FUNCTION "COMANDO USCITE" : VOID
TITLE =COMANDO USCITE
VERSION : 0.1

BEGIN
NETWORK
TITLE =RIPRISTINO EMERGENZA
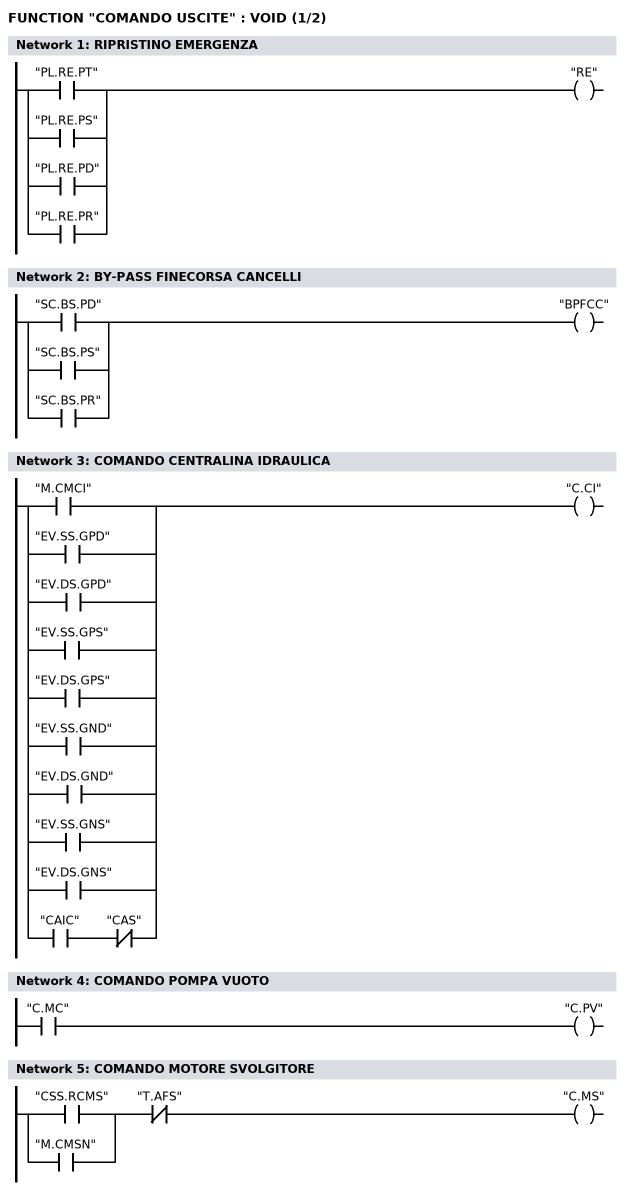
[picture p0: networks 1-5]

      O     "PL.RE.PT";
      O     "PL.RE.PS";
      O     "PL.RE.PD";
      O     "PL.RE.PR";
      =     "RE";
NETWORK
TITLE =BY-PASS FINECORSA CANCELLI

      O     "SC.BS.PD";
      O     "SC.BS.PS";
      O     "SC.BS.PR";
      =     "BPFCC";
NETWORK
TITLE =COMANDO CENTRALINA IDRAULICA

      O     "M.CMCI";
      O     "EV.SS.GPD";
      O     "EV.DS.GPD";
      O     "EV.SS.GPS";
      O     "EV.DS.GPS";
      O     "EV.SS.GND";
      O     "EV.DS.GND";
      O     "EV.SS.GNS";
      O     "EV.DS.GNS";
      O     ;
      U     "CAIC";
      UN    "CAS";
      =     "C.CI";
NETWORK
TITLE =COMANDO POMPA VUOTO

      O     "C.MC";
      =     "C.PV";
NETWORK
TITLE =COMANDO MOTORE SVOLGITORE

      U(    ;
      O     "CSS.RCMS";
      O     "M.CMSN";
      )     ;
      UN    "T.AFS";
      =     "C.MS";
NETWORK
TITLE =COMANDO MOTORE CATENE
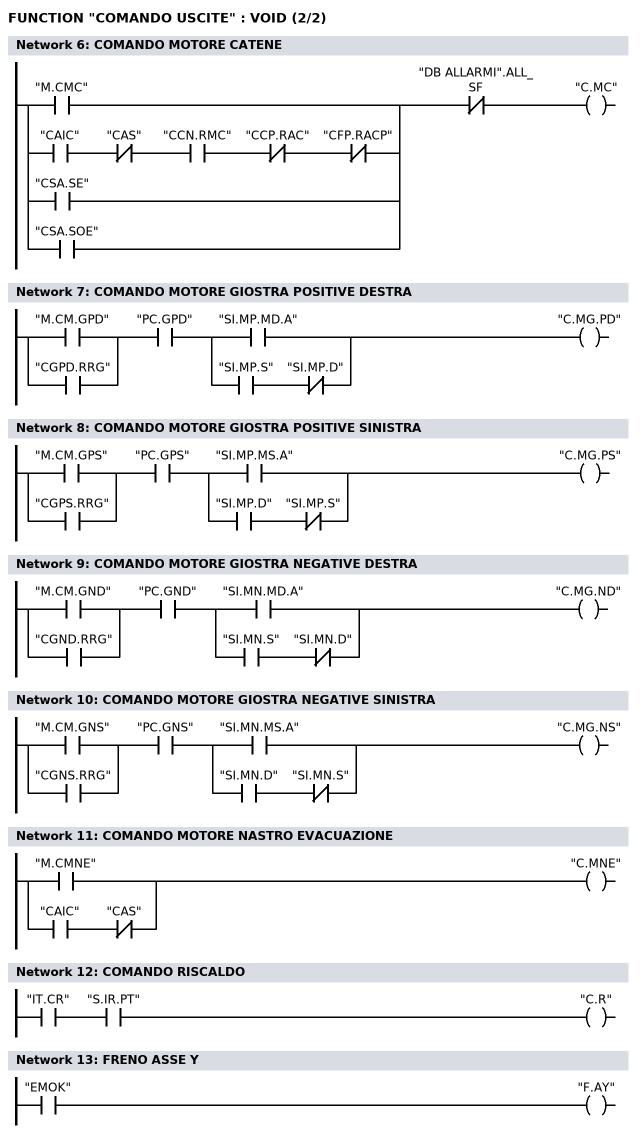
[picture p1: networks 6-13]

      U(    ;
      O     "M.CMC";
      O     ;
      U     "CAIC";
      UN    "CAS";
      U     "CCN.RMC";
      UN    "CCP.RAC";
      UN    "CFP.RACP";
      O     "CSA.SE";
      O     "CSA.SOE";
      )     ;
      UN    "DB ALLARMI".ALL_SF;
      =     "C.MC";
NETWORK
TITLE =COMANDO MOTORE GIOSTRA POSITIVE DESTRA

      U(    ;
      O     "M.CM.GPD";
      O     "CGPD.RRG";
      )     ;
      U     "PC.GPD";
      U(    ;
      O     "SI.MP.MD.A";
      O     ;
      U     "SI.MP.S";
      UN    "SI.MP.D";
      )     ;
      =     "C.MG.PD";
NETWORK
TITLE =COMANDO MOTORE GIOSTRA POSITIVE SINISTRA

      U(    ;
      O     "M.CM.GPS";
      O     "CGPS.RRG";
      )     ;
      U     "PC.GPS";
      U(    ;
      O     "SI.MP.MS.A";
      O     ;
      U     "SI.MP.D";
      UN    "SI.MP.S";
      )     ;
      =     "C.MG.PS";
NETWORK
TITLE =COMANDO MOTORE GIOSTRA NEGATIVE DESTRA

      U(    ;
      O     "M.CM.GND";
      O     "CGND.RRG";
      )     ;
      U     "PC.GND";
      U(    ;
      O     "SI.MN.MD.A";
      O     ;
      U     "SI.MN.S";
      UN    "SI.MN.D";
      )     ;
      =     "C.MG.ND";
NETWORK
TITLE =COMANDO MOTORE GIOSTRA NEGATIVE SINISTRA

      U(    ;
      O     "M.CM.GNS";
      O     "CGNS.RRG";
      )     ;
      U     "PC.GNS";
      U(    ;
      O     "SI.MN.MS.A";
      O     ;
      U     "SI.MN.D";
      UN    "SI.MN.S";
      )     ;
      =     "C.MG.NS";
NETWORK
TITLE =COMANDO MOTORE NASTRO EVACUAZIONE

      O     "M.CMNE";
      O     ;
      U     "CAIC";
      UN    "CAS";
      =     "C.MNE";
NETWORK
TITLE =COMANDO RISCALDO

      U     "IT.CR";
      U     "S.IR.PT";
      =     "C.R";
NETWORK
TITLE =FRENO ASSE Y

      U     "EMOK";
//      UN    "SC.BS.PR"
      =     "F.AY";
NETWORK
TITLE =AGGANCIO FRIZIONE IMBUSTATRICE

      UN(   ;
      O     "M.CAFI";
      O     ;
      U     "CAIC";
      U     "CCP.RAF";
      )     ;
      =     "A.FI";
NETWORK
TITLE =SBLOCCO RIPARI
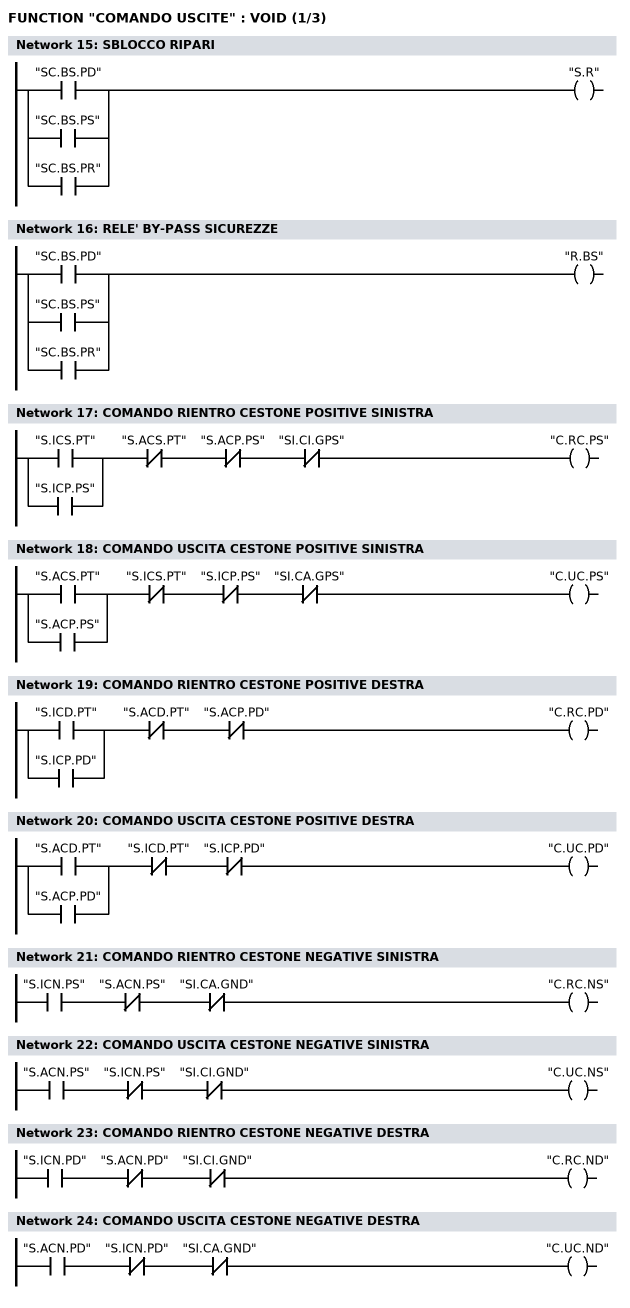
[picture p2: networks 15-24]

      O     "SC.BS.PD";
      O     "SC.BS.PS";
      O     "SC.BS.PR";
      =     "S.R";
NETWORK
TITLE =RELE' BY-PASS SICUREZZE

      O     "SC.BS.PD";
      O     "SC.BS.PS";
      O     "SC.BS.PR";
      =     "R.BS";
NETWORK
TITLE =COMANDO RIENTRO CESTONE POSITIVE SINISTRA

      O     "S.ICS.PT";
      O     "S.ICP.PS";
      UN    "S.ACS.PT";
      UN    "S.ACP.PS";
      UN    "SI.CI.GPS";
      =     "C.RC.PS";
NETWORK
TITLE =COMANDO USCITA CESTONE POSITIVE SINISTRA

      O     "S.ACS.PT";
      O     "S.ACP.PS";
      UN    "S.ICS.PT";
      UN    "S.ICP.PS";
      UN    "SI.CA.GPS";
      =     "C.UC.PS";
NETWORK
TITLE =COMANDO RIENTRO CESTONE POSITIVE DESTRA

      O     "S.ICD.PT";
      O     "S.ICP.PD";
      UN    "S.ACD.PT";
      UN    "S.ACP.PD";
// UN    "SI.CI.GPD"
      =     "C.RC.PD";
NETWORK
TITLE =COMANDO USCITA CESTONE POSITIVE DESTRA

      U     "S.ACD.PT";
      O     "S.ACP.PD";
      UN    "S.ICD.PT";
      UN    "S.ICP.PD";
//  UN    "SI.CA.GPD"
      =     "C.UC.PD";
NETWORK
TITLE =COMANDO RIENTRO CESTONE NEGATIVE SINISTRA

      U     "S.ICN.PS";
      UN    "S.ACN.PS";
      UN    "SI.CA.GND";
      =     "C.RC.NS";
NETWORK
TITLE =COMANDO USCITA CESTONE NEGATIVE SINISTRA

      U     "S.ACN.PS";
      UN    "S.ICN.PS";
      UN    "SI.CI.GND";
      =     "C.UC.NS";
NETWORK
TITLE =COMANDO RIENTRO CESTONE NEGATIVE DESTRA

      U     "S.ICN.PD";
      UN    "S.ACN.PD";
      UN    "SI.CI.GND";
      =     "C.RC.ND";
NETWORK
TITLE =COMANDO USCITA CESTONE NEGATIVE DESTRA

      U     "S.ACN.PD";
      UN    "S.ICN.PD";
      UN    "SI.CA.GND";
      =     "C.UC.ND";
NETWORK
TITLE =COMANDO APERTURA FRENO GIOSTRA POSITIVA DESTRA
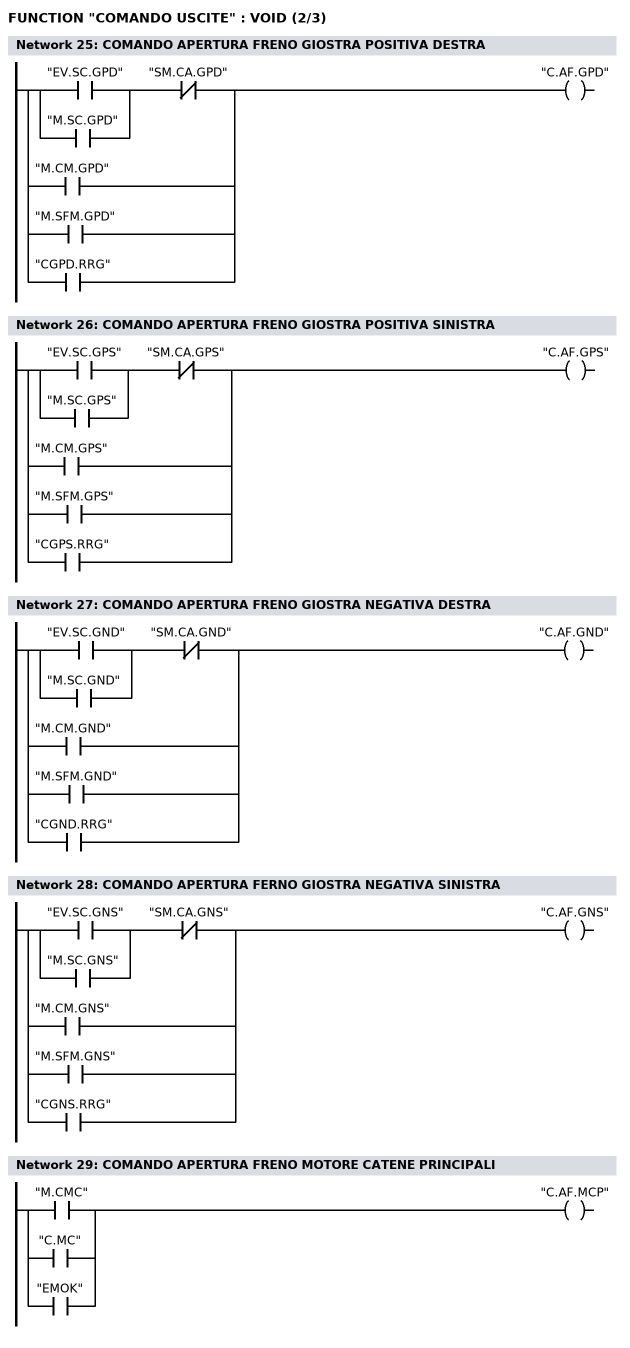
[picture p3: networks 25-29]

      O     "EV.SC.GPD";
      O     "M.SC.GPD";
      UN    "SM.CA.GPD";
      O     ;
      O     "M.CM.GPD";
      O     "M.SFM.GPD";
      O     "CGPD.RRG";
      =     "C.AF.GPD";
NETWORK
TITLE =COMANDO APERTURA FRENO GIOSTRA POSITIVA SINISTRA

      O     "EV.SC.GPS";
      O     "M.SC.GPS";
      UN    "SM.CA.GPS";
      O     ;
      O     "M.CM.GPS";
      O     "M.SFM.GPS";
      O     "CGPS.RRG";
      =     "C.AF.GPS";
NETWORK
TITLE =COMANDO APERTURA FRENO GIOSTRA NEGATIVA DESTRA

      O     "EV.SC.GND";
      O     "M.SC.GND";
      UN    "SM.CA.GND";
      O     ;
      O     "M.CM.GND";
      O     "M.SFM.GND";
      O     "CGND.RRG";
      =     "C.AF.GND";
NETWORK
TITLE =COMANDO APERTURA FERNO GIOSTRA NEGATIVA SINISTRA

      O     "EV.SC.GNS";
      O     "M.SC.GNS";
      UN    "SM.CA.GNS";
      O     ;
      O     "M.CM.GNS";
      O     "M.SFM.GNS";
      O     "CGNS.RRG";
      =     "C.AF.GNS";
NETWORK
TITLE =COMANDO APERTURA FRENO MOTORE CATENE PRINCIPALI

      O     "M.CMC";
      O     "C.MC";
      O     "EMOK";
      =     "C.AF.MCP";
NETWORK
TITLE =COMANDO ABILITAZIONE REGOLATORE ASSE X
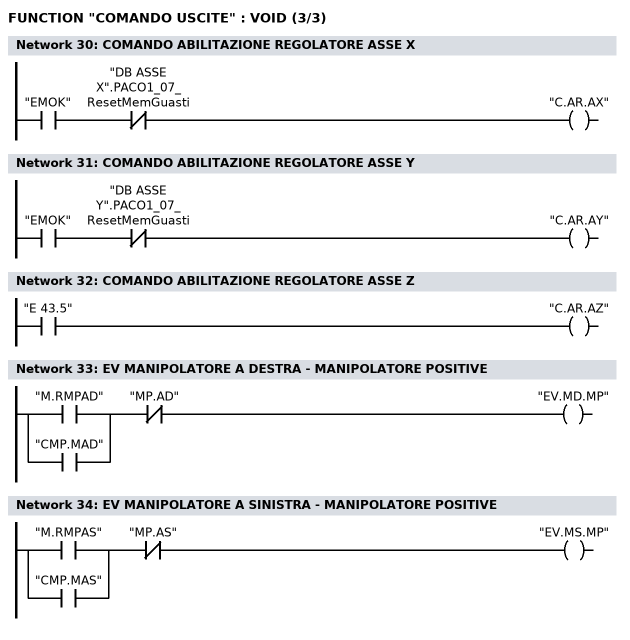
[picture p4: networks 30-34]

      U     "EMOK";
      UN    "DB ASSE X".PACO1_07_ResetMemGuasti;
      =     "C.AR.AX";
NETWORK
TITLE =COMANDO ABILITAZIONE REGOLATORE ASSE Y

      U     "EMOK";
      UN    "DB ASSE Y".PACO1_07_ResetMemGuasti;
      =     "C.AR.AY";
NETWORK
TITLE =COMANDO ABILITAZIONE REGOLATORE ASSE Z

      U     "E      43.5";
      =     "C.AR.AZ";
NETWORK
TITLE =EV MANIPOLATORE A DESTRA - MANIPOLATORE POSITIVE

      O     "M.RMPAD";
      O     "CMP.MAD";
      UN    "MP.AD";
      =     "EV.MD.MP";
NETWORK
TITLE =EV MANIPOLATORE A SINISTRA - MANIPOLATORE POSITIVE

      O     "M.RMPAS";
      O     "CMP.MAS";
      UN    "MP.AS";
      =     "EV.MS.MP";
NETWORK
TITLE =scorta

      CLR   ;
      =     "A      14.2";
NETWORK
TITLE =scorta

      CLR   ;
      =     "A      14.3";
NETWORK
TITLE =EV SALITA MANO DESTRA MANIPOLATORE POSITIVE
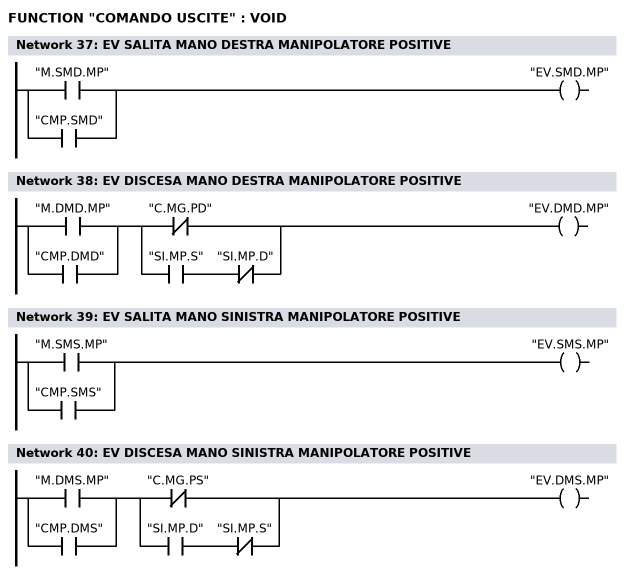
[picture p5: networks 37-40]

      O     "M.SMD.MP";
      O     "CMP.SMD";
      =     "EV.SMD.MP";
NETWORK
TITLE =EV DISCESA MANO DESTRA MANIPOLATORE POSITIVE

      U(    ;
      O     "M.DMD.MP";
      O     "CMP.DMD";
      )     ;
      U(    ;
      ON    "C.MG.PD";
      O     ;
      U     "SI.MP.S";
      UN    "SI.MP.D";
      )     ;
      =     "EV.DMD.MP";
NETWORK
TITLE =EV SALITA MANO SINISTRA MANIPOLATORE POSITIVE

      O     "M.SMS.MP";
      O     "CMP.SMS";
      =     "EV.SMS.MP";
NETWORK
TITLE =EV DISCESA MANO SINISTRA MANIPOLATORE POSITIVE

      U(    ;
      O     "M.DMS.MP";
      O     "CMP.DMS";
      )     ;
      U(    ;
      ON    "C.MG.PS";
      O     ;
      U     "SI.MP.D";
      UN    "SI.MP.S";
      )     ;
      =     "EV.DMS.MP";
NETWORK
TITLE =

      CLR   ;
      =     "A      15.0";
NETWORK
TITLE =

      CLR   ;
      =     "A      15.1";
NETWORK
TITLE =scorta

      CLR   ;
      =     "A      15.2";
NETWORK
TITLE =scorta

      CLR   ;
      =     "A      15.3";
NETWORK
TITLE =LP EMERGENZA
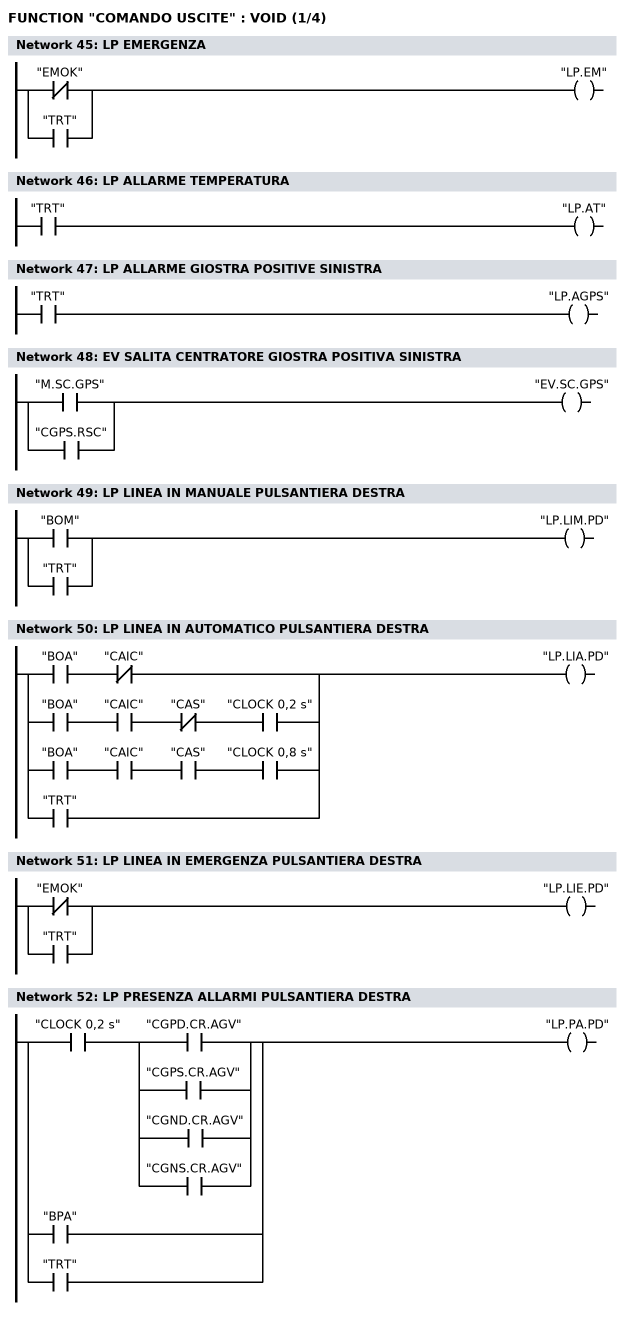
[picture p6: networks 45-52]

      ON    "EMOK";
      O     "TRT";
      =     "LP.EM";
NETWORK
TITLE =LP ALLARME TEMPERATURA

      O     "TRT";
      =     "LP.AT";
NETWORK
TITLE =LP ALLARME GIOSTRA POSITIVE SINISTRA

      O     "TRT";
      =     "LP.AGPS";
NETWORK
TITLE =EV SALITA CENTRATORE GIOSTRA POSITIVA SINISTRA

      O     "M.SC.GPS";
      O     "CGPS.RSC";
      =     "EV.SC.GPS";
NETWORK
TITLE =LP LINEA IN MANUALE PULSANTIERA DESTRA

      O     "BOM";
      O     "TRT";
      =     "LP.LIM.PD";
NETWORK
TITLE =LP LINEA IN AUTOMATICO PULSANTIERA DESTRA

      U     "BOA";
      UN    "CAIC";
      O     ;
      U     "BOA";
      U     "CAIC";
      UN    "CAS";
      U     "CLOCK 0,2 s";
      O     ;
      U     "BOA";
      U     "CAIC";
      U     "CAS";
      U     "CLOCK 0,8 s";
      O     "TRT";
      =     "LP.LIA.PD";
NETWORK
TITLE =LP LINEA IN EMERGENZA PULSANTIERA DESTRA

      ON    "EMOK";
      O     "TRT";
      =     "LP.LIE.PD";
NETWORK
TITLE =LP PRESENZA ALLARMI PULSANTIERA DESTRA

      U     "CLOCK 0,2 s";
      U(    ;
      O     "CGPD.CR.AGV";
      O     "CGPS.CR.AGV";
      O     "CGND.CR.AGV";
      O     "CGNS.CR.AGV";
      )     ;
      O     "BPA";
      O     "TRT";
      =     "LP.PA.PD";
NETWORK
TITLE =LP MARCIA MOTORE GIOSTRA PULSANTIERA DESTRA
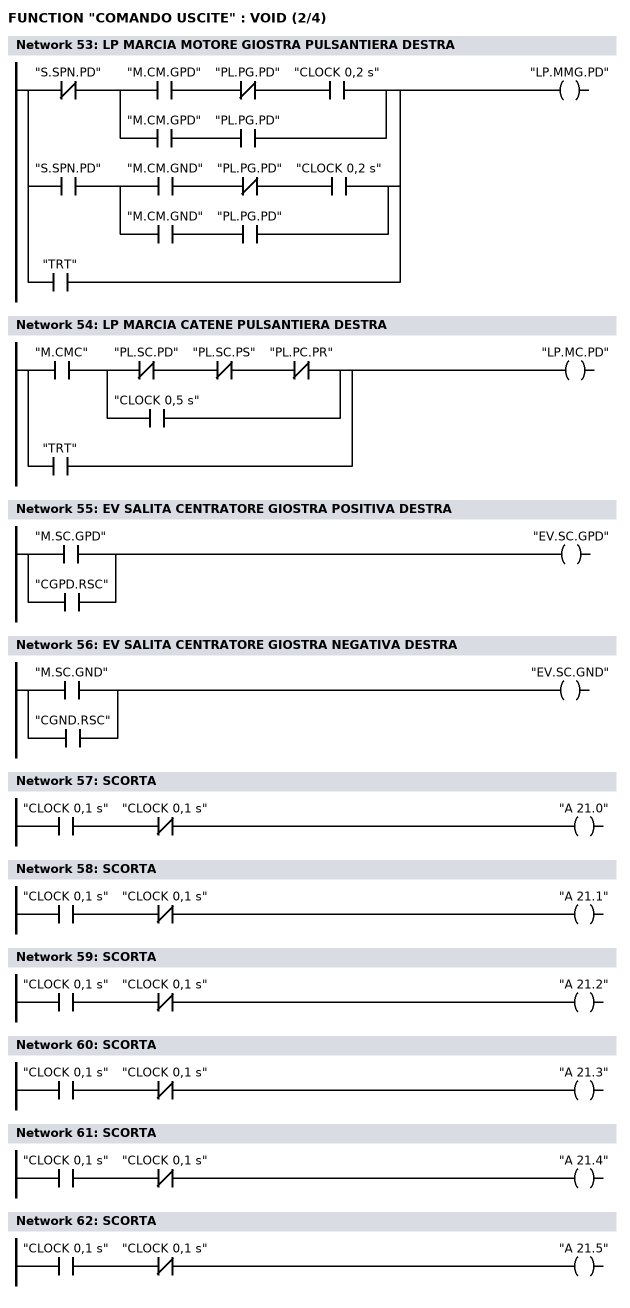
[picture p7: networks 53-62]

      UN    "S.SPN.PD";
      U(    ;
      U     "M.CM.GPD";
      UN    "PL.PG.PD";
      U     "CLOCK 0,2 s";
      O     ;
      U     "M.CM.GPD";
      U     "PL.PG.PD";
      )     ;
      O     ;
      U     "S.SPN.PD";
      U(    ;
      U     "M.CM.GND";
      UN    "PL.PG.PD";
      U     "CLOCK 0,2 s";
      O     ;
      U     "M.CM.GND";
      U     "PL.PG.PD";
      )     ;
      O     "TRT";
      =     "LP.MMG.PD";
NETWORK
TITLE =LP MARCIA CATENE PULSANTIERA DESTRA

      U     "M.CMC";
      U(    ;
      UN    "PL.SC.PD";
      UN    "PL.SC.PS";
      UN    "PL.PC.PR";
      O     "CLOCK 0,5 s";
      )     ;
      O     "TRT";
      =     "LP.MC.PD";
NETWORK
TITLE =EV SALITA CENTRATORE GIOSTRA POSITIVA DESTRA

      O     "M.SC.GPD";
      O     "CGPD.RSC";
      =     "EV.SC.GPD";
NETWORK
TITLE =EV SALITA CENTRATORE GIOSTRA NEGATIVA DESTRA

      O     "M.SC.GND";
      O     "CGND.RSC";
      =     "EV.SC.GND";
NETWORK
TITLE =SCORTA

      U     "CLOCK 0,1 s";
      UN    "CLOCK 0,1 s";
      =     "A      21.0";
NETWORK
TITLE =SCORTA

      U     "CLOCK 0,1 s";
      UN    "CLOCK 0,1 s";
      =     "A      21.1";
NETWORK
TITLE =SCORTA

      U     "CLOCK 0,1 s";
      UN    "CLOCK 0,1 s";
      =     "A      21.2";
NETWORK
TITLE =SCORTA

      U     "CLOCK 0,1 s";
      UN    "CLOCK 0,1 s";
      =     "A      21.3";
NETWORK
TITLE =SCORTA

      U     "CLOCK 0,1 s";
      UN    "CLOCK 0,1 s";
      =     "A      21.4";
NETWORK
TITLE =SCORTA

      U     "CLOCK 0,1 s";
      UN    "CLOCK 0,1 s";
      =     "A      21.5";
NETWORK
TITLE =SCORTA
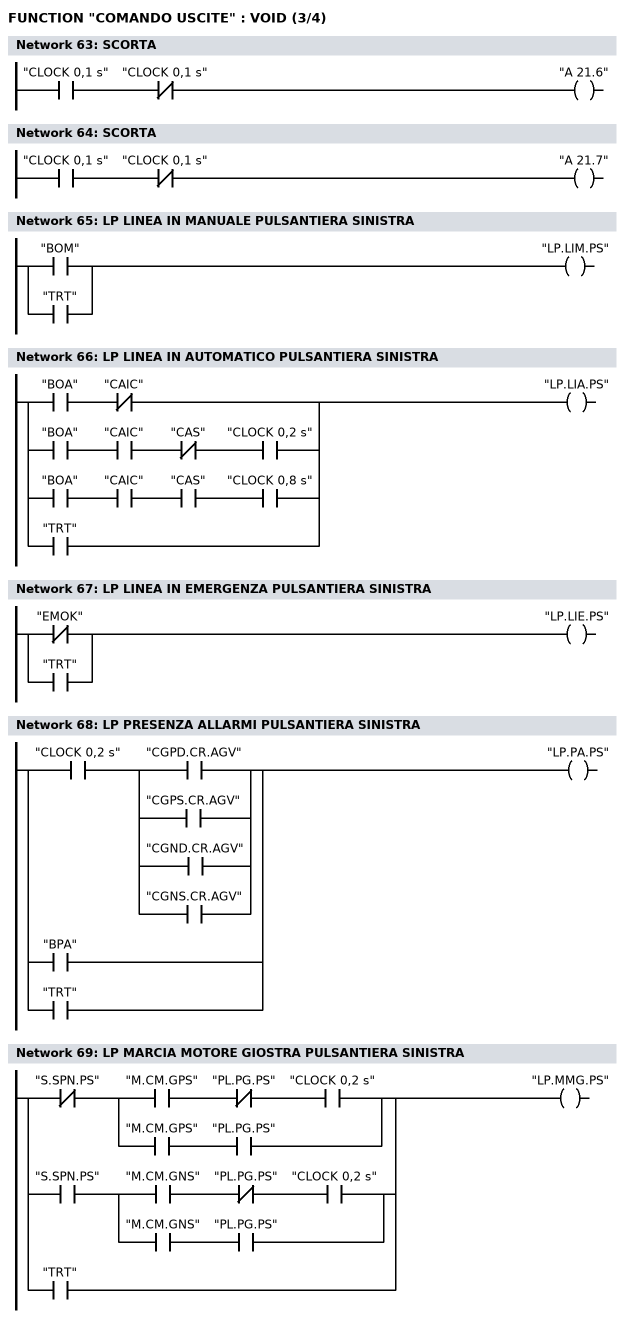
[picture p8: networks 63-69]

      U     "CLOCK 0,1 s";
      UN    "CLOCK 0,1 s";
      =     "A      21.6";
NETWORK
TITLE =SCORTA

      U     "CLOCK 0,1 s";
      UN    "CLOCK 0,1 s";
      =     "A      21.7";
NETWORK
TITLE =LP LINEA IN MANUALE PULSANTIERA SINISTRA

      O     "BOM";
      O     "TRT";
      =     "LP.LIM.PS";
NETWORK
TITLE =LP LINEA IN AUTOMATICO PULSANTIERA SINISTRA

      U     "BOA";
      UN    "CAIC";
      O     ;
      U     "BOA";
      U     "CAIC";
      UN    "CAS";
      U     "CLOCK 0,2 s";
      O     ;
      U     "BOA";
      U     "CAIC";
      U     "CAS";
      U     "CLOCK 0,8 s";
      O     "TRT";
      =     "LP.LIA.PS";
NETWORK
TITLE =LP LINEA IN EMERGENZA PULSANTIERA SINISTRA

      ON    "EMOK";
      O     "TRT";
      =     "LP.LIE.PS";
NETWORK
TITLE =LP PRESENZA ALLARMI PULSANTIERA SINISTRA

      U     "CLOCK 0,2 s";
      U(    ;
      O     "CGPD.CR.AGV";
      O     "CGPS.CR.AGV";
      O     "CGND.CR.AGV";
      O     "CGNS.CR.AGV";
      )     ;
      O     "BPA";
      O     "TRT";
      =     "LP.PA.PS";
NETWORK
TITLE =LP MARCIA MOTORE GIOSTRA PULSANTIERA SINISTRA

      UN    "S.SPN.PS";
      U(    ;
      U     "M.CM.GPS";
      UN    "PL.PG.PS";
      U     "CLOCK 0,2 s";
      O     ;
      U     "M.CM.GPS";
      U     "PL.PG.PS";
      )     ;
      O     ;
      U     "S.SPN.PS";
      U(    ;
      U     "M.CM.GNS";
      UN    "PL.PG.PS";
      U     "CLOCK 0,2 s";
      O     ;
      U     "M.CM.GNS";
      U     "PL.PG.PS";
      )     ;
      O     "TRT";
      =     "LP.MMG.PS";
NETWORK
TITLE =LP MARCIA CATENE PULSANTIERA SINISTRA
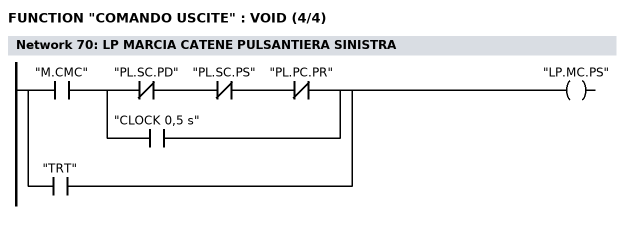
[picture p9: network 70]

      U     "M.CMC";
      U(    ;
      UN    "PL.SC.PD";
      UN    "PL.SC.PS";
      UN    "PL.PC.PR";
      O     "CLOCK 0,5 s";
      )     ;
      O     "TRT";
      =     "LP.MC.PS";
NETWORK
TITLE =LP ALLARME GIOSTRA POSITIVE DESTRA

      CLR   ;
      O     "TRT";
      =     "LP.AGPD";
NETWORK
TITLE =SCORTA

      CLR   ;
      =     "A      26.7";
NETWORK
TITLE =SCORTA

      CLR   ;
      =     "A      27.0";
NETWORK
TITLE =SCORTA

      CLR   ;
      =     "A      27.1";
NETWORK
TITLE =SCORTA

      CLR   ;
      =     "A      27.2";
NETWORK
TITLE =SCORTA

      CLR   ;
      =     "A      27.3";
NETWORK
TITLE =SCORTA

      CLR   ;
      =     "A      27.4";
NETWORK
TITLE =SCORTA

      CLR   ;
      =     "A      27.5";
NETWORK
TITLE =SCORTA

      CLR   ;
      =     "A      27.6";
NETWORK
TITLE =SCORTA

      CLR   ;
      =     "A      27.7";
NETWORK
TITLE =EV MANIPOLATORE A DESTRA - MANIPOLATORE NEGATIVE
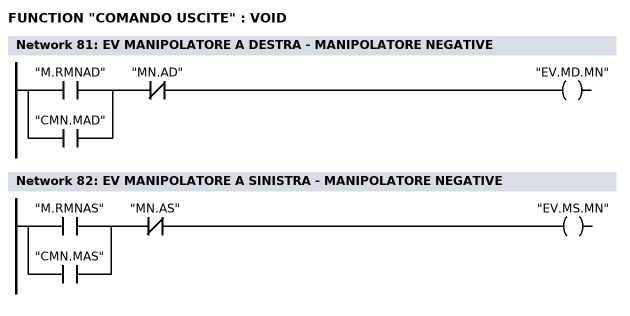
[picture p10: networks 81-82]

      U     "M.RMNAD";
      O     "CMN.MAD";
      UN    "MN.AD";
      =     "EV.MD.MN";
NETWORK
TITLE =EV MANIPOLATORE A SINISTRA - MANIPOLATORE NEGATIVE

      U     "M.RMNAS";
      O     "CMN.MAS";
      UN    "MN.AS";
      =     "EV.MS.MN";
NETWORK
TITLE =scorta

      CLR   ;
      =     "A      28.2";
NETWORK
TITLE =scorta

      CLR   ;
      =     "A      28.3";
NETWORK
TITLE =EV SALITA MANO DESTRA MANIPOLATORE NEGATIVE
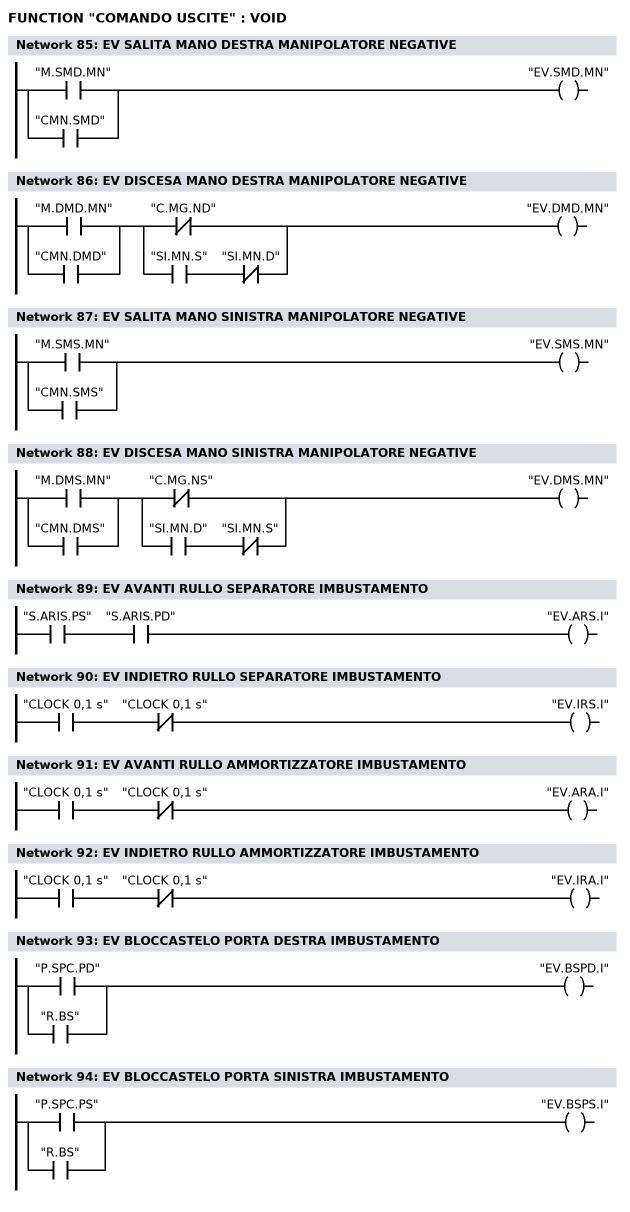
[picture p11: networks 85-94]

      O     "M.SMD.MN";
      O     "CMN.SMD";
      =     "EV.SMD.MN";
NETWORK
TITLE =EV DISCESA MANO DESTRA MANIPOLATORE NEGATIVE

      U(    ;
      O     "M.DMD.MN";
      O     "CMN.DMD";
      )     ;
      U(    ;
      ON    "C.MG.ND";
      O     ;
      U     "SI.MN.S";
      UN    "SI.MN.D";
      )     ;
      =     "EV.DMD.MN";
NETWORK
TITLE =EV SALITA MANO SINISTRA MANIPOLATORE NEGATIVE

      O     "M.SMS.MN";
      O     "CMN.SMS";
      =     "EV.SMS.MN";
NETWORK
TITLE =EV DISCESA MANO SINISTRA MANIPOLATORE NEGATIVE

      U(    ;
      O     "M.DMS.MN";
      O     "CMN.DMS";
      )     ;
      U(    ;
      ON    "C.MG.NS";
      O     ;
      U     "SI.MN.D";
      UN    "SI.MN.S";
      )     ;
      =     "EV.DMS.MN";
NETWORK
TITLE =EV AVANTI RULLO SEPARATORE IMBUSTAMENTO

      U     "S.ARIS.PS";
      U     "S.ARIS.PD";
      =     "EV.ARS.I";
NETWORK
TITLE =EV INDIETRO RULLO SEPARATORE IMBUSTAMENTO

      U     "CLOCK 0,1 s";
      UN    "CLOCK 0,1 s";
      =     "EV.IRS.I";
NETWORK
TITLE =EV AVANTI RULLO AMMORTIZZATORE IMBUSTAMENTO

      U     "CLOCK 0,1 s";
      UN    "CLOCK 0,1 s";
      =     "EV.ARA.I";
NETWORK
TITLE =EV INDIETRO RULLO AMMORTIZZATORE IMBUSTAMENTO

      U     "CLOCK 0,1 s";
      UN    "CLOCK 0,1 s";
      =     "EV.IRA.I";
NETWORK
TITLE =EV BLOCCASTELO PORTA DESTRA IMBUSTAMENTO

      O     "P.SPC.PD";
      O     "R.BS";
      =     "EV.BSPD.I";
NETWORK
TITLE =EV BLOCCASTELO PORTA SINISTRA IMBUSTAMENTO

      O     "P.SPC.PS";
      O     "R.BS";
      =     "EV.BSPS.I";
NETWORK
TITLE =

      CLR   ;
      =     "A      29.6";
NETWORK
TITLE =

      CLR   ;
      =     "A      29.7";
NETWORK
TITLE =EV SALITA SOLLEVATORE GIOSTRA POSITIVE SINISTRA
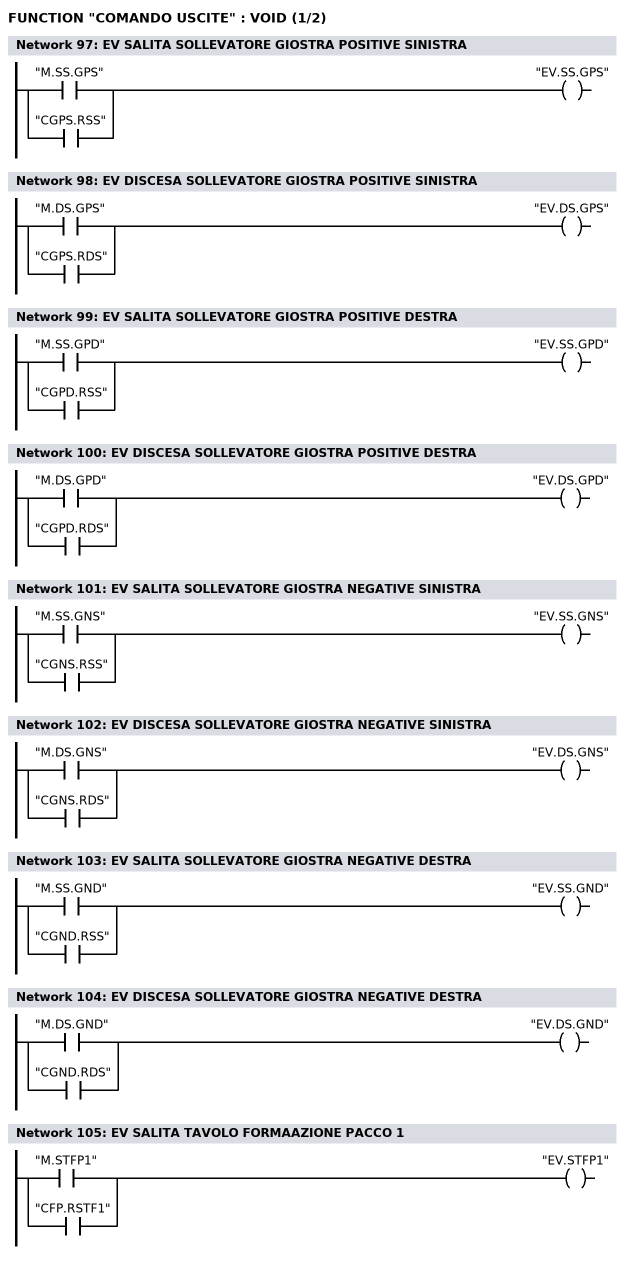
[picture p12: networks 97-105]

      O     "M.SS.GPS";
      O     "CGPS.RSS";
      =     "EV.SS.GPS";
NETWORK
TITLE =EV DISCESA SOLLEVATORE GIOSTRA POSITIVE SINISTRA

      O     "M.DS.GPS";
      O     "CGPS.RDS";
      =     "EV.DS.GPS";
NETWORK
TITLE =EV SALITA SOLLEVATORE GIOSTRA POSITIVE DESTRA

      O     "M.SS.GPD";
      O     "CGPD.RSS";
      =     "EV.SS.GPD";
NETWORK
TITLE =EV DISCESA SOLLEVATORE GIOSTRA POSITIVE DESTRA

      O     "M.DS.GPD";
      O     "CGPD.RDS";
      =     "EV.DS.GPD";
NETWORK
TITLE =EV SALITA SOLLEVATORE GIOSTRA NEGATIVE SINISTRA

      O     "M.SS.GNS";
      O     "CGNS.RSS";
      =     "EV.SS.GNS";
NETWORK
TITLE =EV DISCESA SOLLEVATORE GIOSTRA NEGATIVE SINISTRA

      O     "M.DS.GNS";
      O     "CGNS.RDS";
      =     "EV.DS.GNS";
NETWORK
TITLE =EV SALITA SOLLEVATORE GIOSTRA NEGATIVE DESTRA

      O     "M.SS.GND";
      O     "CGND.RSS";
      =     "EV.SS.GND";
NETWORK
TITLE =EV DISCESA SOLLEVATORE GIOSTRA NEGATIVE DESTRA

      O     "M.DS.GND";
      O     "CGND.RDS";
      =     "EV.DS.GND";
NETWORK
TITLE =EV SALITA TAVOLO FORMAAZIONE PACCO 1

      O     "M.STFP1";
      O     "CFP.RSTF1";
      =     "EV.STFP1";
NETWORK
TITLE =EV DISCESA TAVOLO FORMAAZIONE PACCO 1
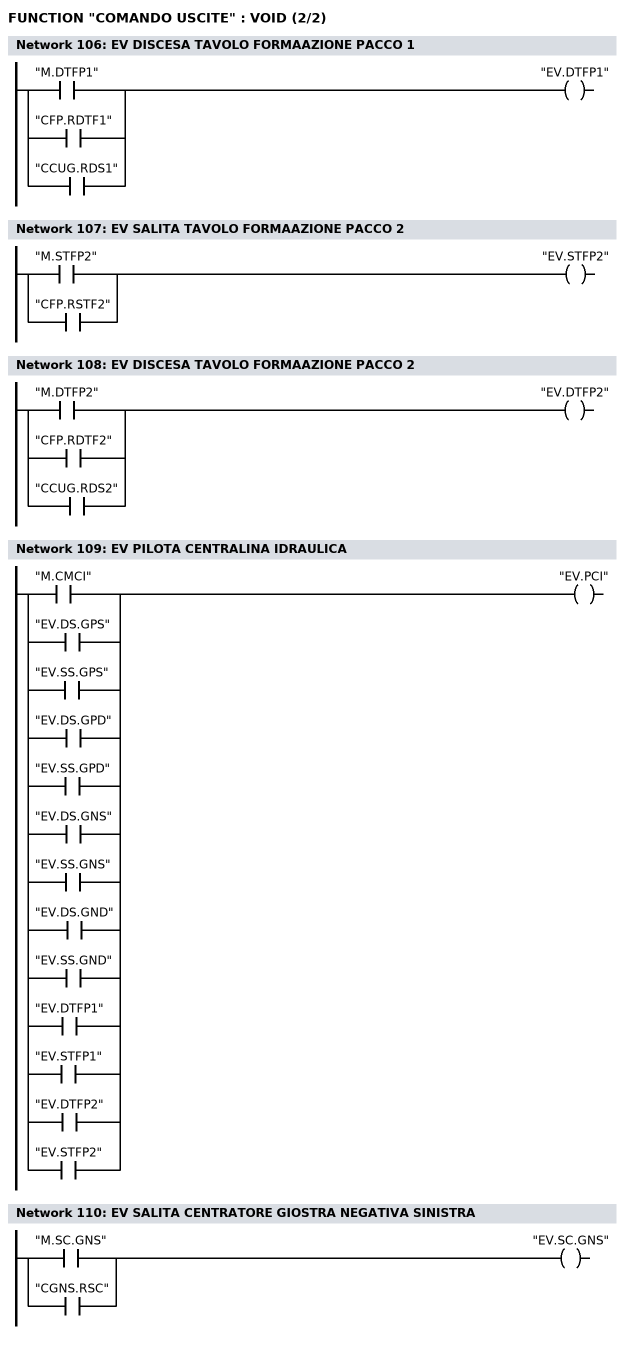
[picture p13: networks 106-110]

      O     "M.DTFP1";
      O     "CFP.RDTF1";
      O     "CCUG.RDS1";
      =     "EV.DTFP1";
NETWORK
TITLE =EV SALITA TAVOLO FORMAAZIONE PACCO 2

      O     "M.STFP2";
      O     "CFP.RSTF2";
      =     "EV.STFP2";
NETWORK
TITLE =EV DISCESA TAVOLO FORMAAZIONE PACCO 2

      O     "M.DTFP2";
      O     "CFP.RDTF2";
      O     "CCUG.RDS2";
      =     "EV.DTFP2";
NETWORK
TITLE =EV PILOTA CENTRALINA IDRAULICA

      O     "M.CMCI";
      O     "EV.DS.GPS";
      O     "EV.SS.GPS";
      O     "EV.DS.GPD";
      O     "EV.SS.GPD";
      O     "EV.DS.GNS";
      O     "EV.SS.GNS";
      O     "EV.DS.GND";
      O     "EV.SS.GND";
      O     "EV.DTFP1";
      O     "EV.STFP1";
      O     "EV.DTFP2";
      O     "EV.STFP2";
      =     "EV.PCI";
NETWORK
TITLE =EV SALITA CENTRATORE GIOSTRA NEGATIVA SINISTRA

      O     "M.SC.GNS";
      O     "CGNS.RSC";
      =     "EV.SC.GNS";
NETWORK
TITLE =scorta

      CLR   ;
      =     "A      31.6";
NETWORK
TITLE =scorta

      CLR   ;
      =     "A      31.7";
NETWORK
TITLE =EV CHIUSURA ARRESTO PACCO 1
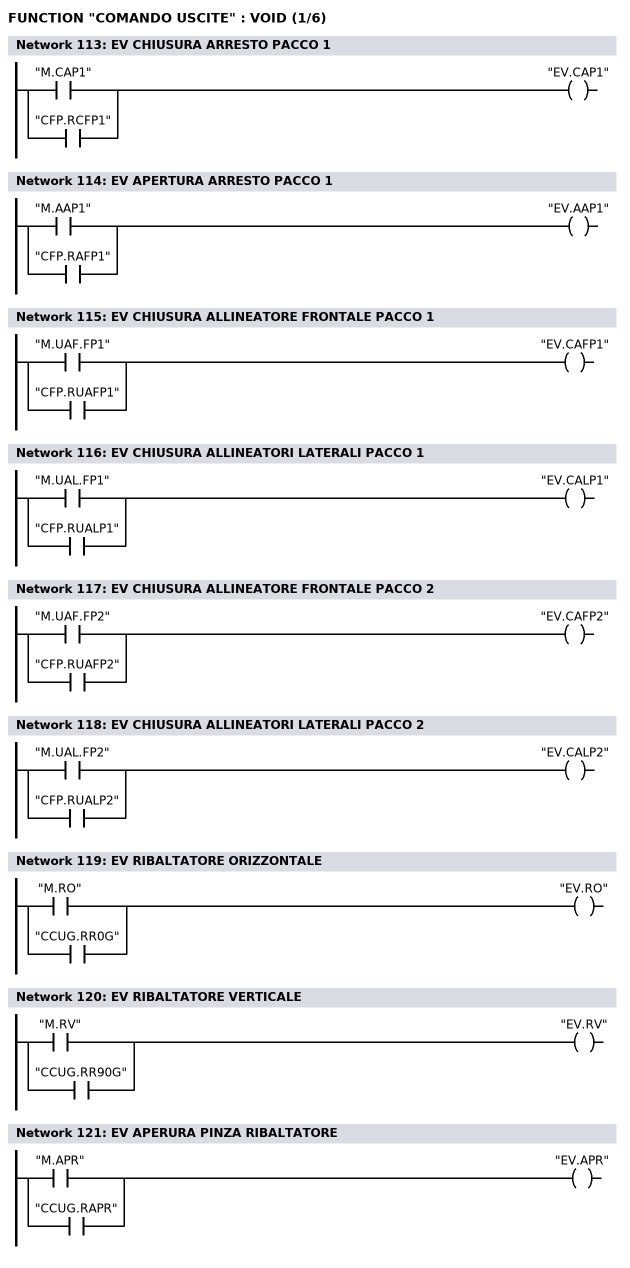
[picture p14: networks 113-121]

      O     "M.CAP1";
      O     "CFP.RCFP1";
      =     "EV.CAP1";
NETWORK
TITLE =EV APERTURA ARRESTO PACCO 1

      O     "M.AAP1";
      O     "CFP.RAFP1";
      =     "EV.AAP1";
NETWORK
TITLE =EV CHIUSURA ALLINEATORE FRONTALE PACCO 1

      O     "M.UAF.FP1";
      O     "CFP.RUAFP1";
      =     "EV.CAFP1";
NETWORK
TITLE =EV CHIUSURA ALLINEATORI LATERALI PACCO 1

      O     "M.UAL.FP1";
      O     "CFP.RUALP1";
      =     "EV.CALP1";
NETWORK
TITLE =EV CHIUSURA ALLINEATORE FRONTALE PACCO 2

      O     "M.UAF.FP2";
      O     "CFP.RUAFP2";
      =     "EV.CAFP2";
NETWORK
TITLE =EV CHIUSURA ALLINEATORI LATERALI PACCO 2

      O     "M.UAL.FP2";
      O     "CFP.RUALP2";
      =     "EV.CALP2";
NETWORK
TITLE =EV RIBALTATORE ORIZZONTALE

      O     "M.RO";
      O     "CCUG.RR0G";
      =     "EV.RO";
NETWORK
TITLE =EV RIBALTATORE VERTICALE

      O     "M.RV";
      O     "CCUG.RR90G";
      =     "EV.RV";
NETWORK
TITLE =EV APERURA PINZA RIBALTATORE

      O     "M.APR";
      O     "CCUG.RAPR";
      =     "EV.APR";
NETWORK
TITLE =EV CHIUSURA PINZA RIBALTATORE
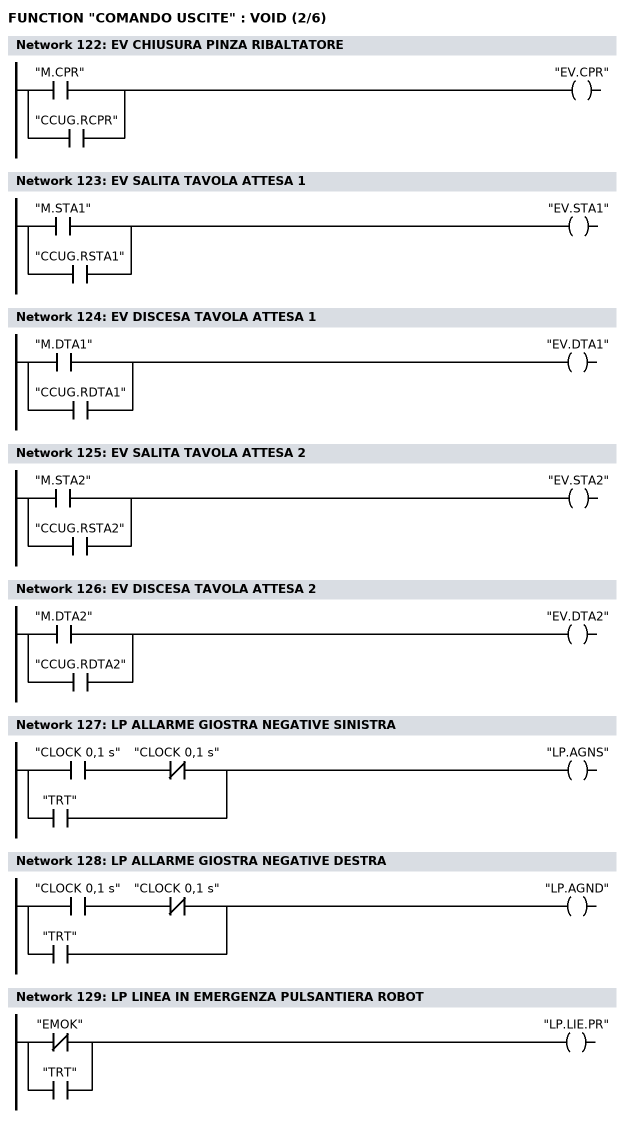
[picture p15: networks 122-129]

      O     "M.CPR";
      O     "CCUG.RCPR";
      =     "EV.CPR";
NETWORK
TITLE =EV SALITA TAVOLA ATTESA 1

      O     "M.STA1";
      O     "CCUG.RSTA1";
      =     "EV.STA1";
NETWORK
TITLE =EV DISCESA TAVOLA ATTESA 1

      O     "M.DTA1";
      O     "CCUG.RDTA1";
      =     "EV.DTA1";
NETWORK
TITLE =EV SALITA TAVOLA ATTESA 2

      O     "M.STA2";
      O     "CCUG.RSTA2";
      =     "EV.STA2";
NETWORK
TITLE =EV DISCESA TAVOLA ATTESA 2

      O     "M.DTA2";
      O     "CCUG.RDTA2";
      =     "EV.DTA2";
NETWORK
TITLE =LP ALLARME GIOSTRA NEGATIVE SINISTRA

      U     "CLOCK 0,1 s";
      UN    "CLOCK 0,1 s";
      O     "TRT";
      =     "LP.AGNS";
NETWORK
TITLE =LP ALLARME GIOSTRA NEGATIVE DESTRA

      U     "CLOCK 0,1 s";
      UN    "CLOCK 0,1 s";
      O     "TRT";
      =     "LP.AGND";
NETWORK
TITLE =LP LINEA IN EMERGENZA PULSANTIERA ROBOT

      ON    "EMOK";
      O     "TRT";
      =     "LP.LIE.PR";
NETWORK
TITLE =LP PRESENZA ALLARMI PULSANTIERA ROBOT
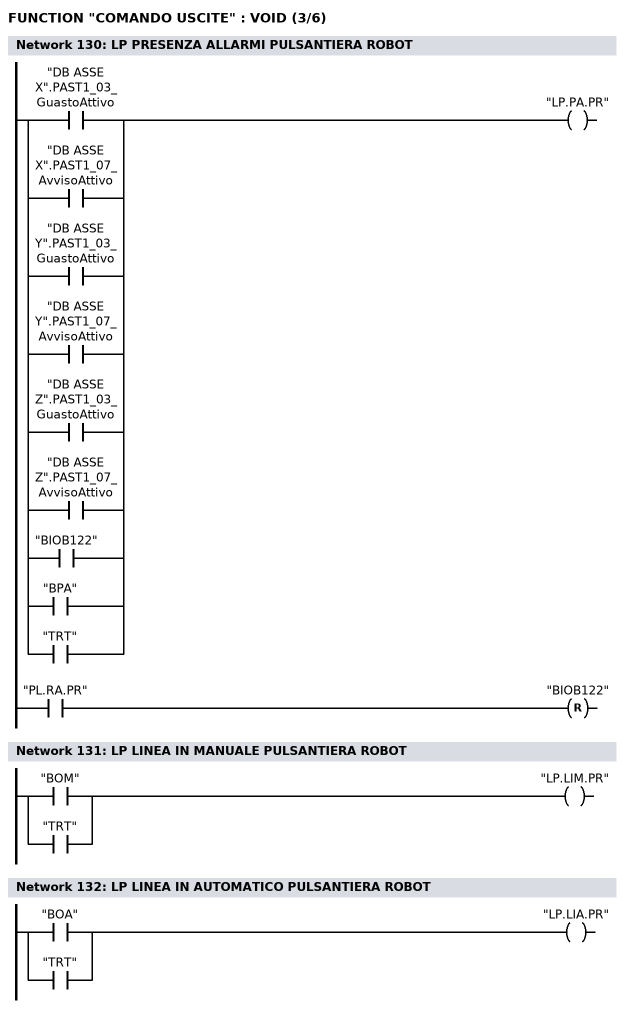
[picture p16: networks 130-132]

      O     "DB ASSE X".PAST1_03_GuastoAttivo;
      O     "DB ASSE X".PAST1_07_AvvisoAttivo;
      O     "DB ASSE Y".PAST1_03_GuastoAttivo;
      O     "DB ASSE Y".PAST1_07_AvvisoAttivo;
      O     "DB ASSE Z".PAST1_03_GuastoAttivo;
      O     "DB ASSE Z".PAST1_07_AvvisoAttivo;
      O     "BIOB122";
      O     "BPA";
      O     "TRT";
      =     "LP.PA.PR";
//__________
      U     "PL.RA.PR";
      R     "BIOB122";
NETWORK
TITLE =LP LINEA IN MANUALE PULSANTIERA ROBOT

      O     "BOM";
      O     "TRT";
      =     "LP.LIM.PR";
NETWORK
TITLE =LP LINEA IN AUTOMATICO PULSANTIERA ROBOT

      O     "BOA";
      O     "TRT";
      =     "LP.LIA.PR";
NETWORK
TITLE =LP LINEA IN JOG-REF PULSANTIERA ROBOT
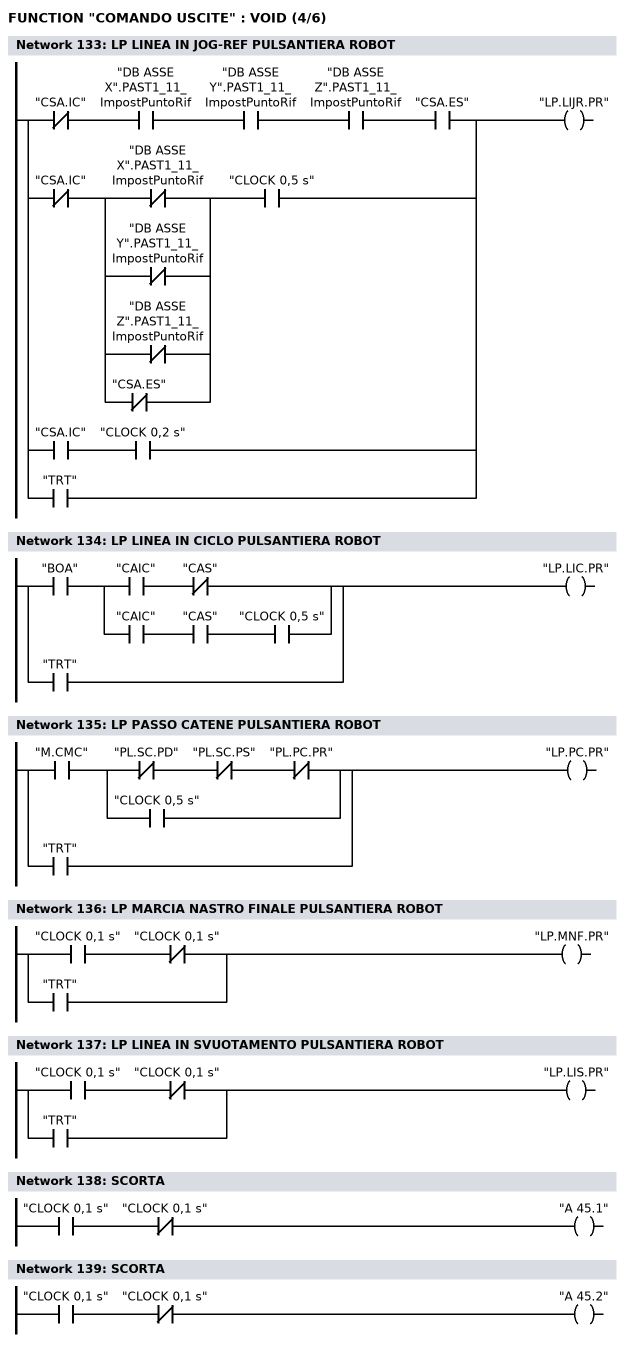
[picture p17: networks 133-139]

      UN    "CSA.IC";
      U     "DB ASSE X".PAST1_11_ImpostPuntoRif;
      U     "DB ASSE Y".PAST1_11_ImpostPuntoRif;
      U     "DB ASSE Z".PAST1_11_ImpostPuntoRif;
      U     "CSA.ES";
      O     ;
      UN    "CSA.IC";
      U(    ;
      ON    "DB ASSE X".PAST1_11_ImpostPuntoRif;
      ON    "DB ASSE Y".PAST1_11_ImpostPuntoRif;
      ON    "DB ASSE Z".PAST1_11_ImpostPuntoRif;
      ON    "CSA.ES";
      )     ;
      U     "CLOCK 0,5 s";
      O     ;
      U     "CSA.IC";
      U     "CLOCK 0,2 s";
      O     "TRT";
      =     "LP.LIJR.PR";
NETWORK
TITLE =LP LINEA IN CICLO PULSANTIERA ROBOT

      U     "BOA";
      U(    ;
      U     "CAIC";
      UN    "CAS";
      O     ;
      U     "CAIC";
      U     "CAS";
      U     "CLOCK 0,5 s";
      )     ;
      O     "TRT";
      =     "LP.LIC.PR";
NETWORK
TITLE =LP PASSO CATENE PULSANTIERA ROBOT

      U     "M.CMC";
      U(    ;
      UN    "PL.SC.PD";
      UN    "PL.SC.PS";
      UN    "PL.PC.PR";
      O     "CLOCK 0,5 s";
      )     ;
      O     "TRT";
      =     "LP.PC.PR";
NETWORK
TITLE =LP MARCIA NASTRO FINALE PULSANTIERA ROBOT

      U     "CLOCK 0,1 s";
      UN    "CLOCK 0,1 s";
      O     "TRT";
      =     "LP.MNF.PR";
NETWORK
TITLE =LP LINEA IN SVUOTAMENTO PULSANTIERA ROBOT

      U     "CLOCK 0,1 s";
      UN    "CLOCK 0,1 s";
      O     "TRT";
      =     "LP.LIS.PR";
NETWORK
TITLE =SCORTA

      U     "CLOCK 0,1 s";
      UN    "CLOCK 0,1 s";
      =     "A      45.1";
NETWORK
TITLE =SCORTA

      U     "CLOCK 0,1 s";
      UN    "CLOCK 0,1 s";
      =     "A      45.2";
NETWORK
TITLE =SCORTA
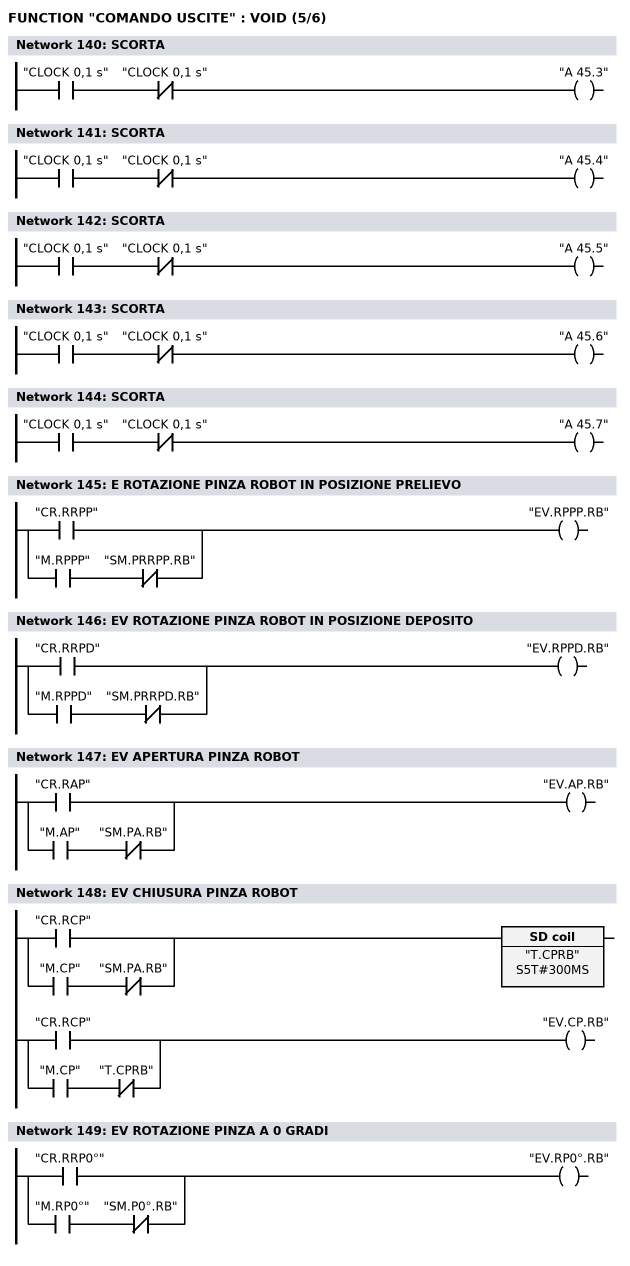
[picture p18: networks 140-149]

      U     "CLOCK 0,1 s";
      UN    "CLOCK 0,1 s";
      =     "A      45.3";
NETWORK
TITLE =SCORTA

      U     "CLOCK 0,1 s";
      UN    "CLOCK 0,1 s";
      =     "A      45.4";
NETWORK
TITLE =SCORTA

      U     "CLOCK 0,1 s";
      UN    "CLOCK 0,1 s";
      =     "A      45.5";
NETWORK
TITLE =SCORTA

      U     "CLOCK 0,1 s";
      UN    "CLOCK 0,1 s";
      =     "A      45.6";
NETWORK
TITLE =SCORTA

      U     "CLOCK 0,1 s";
      UN    "CLOCK 0,1 s";
      =     "A      45.7";
NETWORK
TITLE =E ROTAZIONE PINZA ROBOT IN POSIZIONE PRELIEVO

      O     "CR.RRPP";
      O     ;
      U     "M.RPPP";
      UN    "SM.PRRPP.RB";
      =     "EV.RPPP.RB";
NETWORK
TITLE =EV ROTAZIONE PINZA ROBOT IN POSIZIONE DEPOSITO

      O     "CR.RRPD";
      O     ;
      U     "M.RPPD";
      UN    "SM.PRRPD.RB";
      =     "EV.RPPD.RB";
NETWORK
TITLE =EV APERTURA PINZA ROBOT

      O     "CR.RAP";
      O     ;
      U     "M.AP";
      UN    "SM.PA.RB";
      =     "EV.AP.RB";
NETWORK
TITLE =EV CHIUSURA PINZA ROBOT

      U     "CR.RCP";
      O     ;
      U     "M.CP";
      UN    "SM.PA.RB";
      L     S5T#300MS;
      SE    "T.CPRB";
//-------------------------
      U     "CR.RCP";
      O     ;
      U     "M.CP";
      UN    "T.CPRB";
      =     "EV.CP.RB";

NETWORK
TITLE =EV ROTAZIONE PINZA A 0 GRADI

      O     "CR.RRP0°";
      O     ;
      U     "M.RP0°";
      UN    "SM.P0°.RB";
      =     "EV.RP0°.RB";
NETWORK
TITLE =EV ROTAZIONE PINZA A 180 GRADI
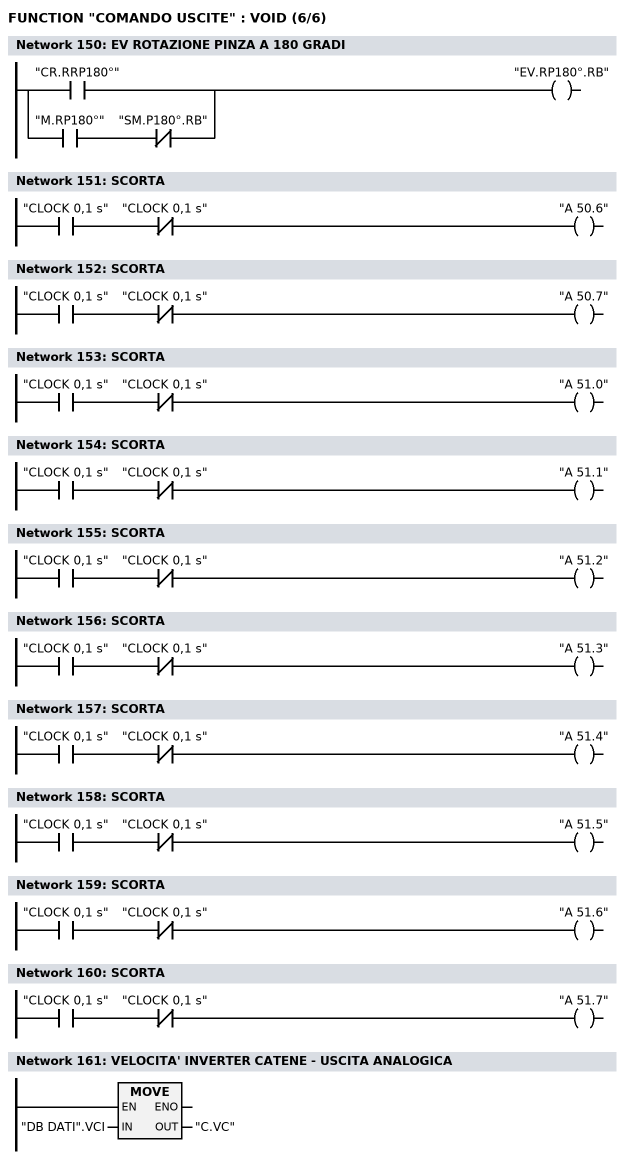
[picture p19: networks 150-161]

      O     "CR.RRP180°";
      O     ;
      U     "M.RP180°";
      UN    "SM.P180°.RB";
      =     "EV.RP180°.RB";
NETWORK
TITLE =SCORTA

      U     "CLOCK 0,1 s";
      UN    "CLOCK 0,1 s";
      =     "A      50.6";
NETWORK
TITLE =SCORTA

      U     "CLOCK 0,1 s";
      UN    "CLOCK 0,1 s";
      =     "A      50.7";
NETWORK
TITLE =SCORTA

      U     "CLOCK 0,1 s";
      UN    "CLOCK 0,1 s";
      =     "A      51.0";
NETWORK
TITLE =SCORTA

      U     "CLOCK 0,1 s";
      UN    "CLOCK 0,1 s";
      =     "A      51.1";
NETWORK
TITLE =SCORTA

      U     "CLOCK 0,1 s";
      UN    "CLOCK 0,1 s";
      =     "A      51.2";
NETWORK
TITLE =SCORTA

      U     "CLOCK 0,1 s";
      UN    "CLOCK 0,1 s";
      =     "A      51.3";
NETWORK
TITLE =SCORTA

      U     "CLOCK 0,1 s";
      UN    "CLOCK 0,1 s";
      =     "A      51.4";
NETWORK
TITLE =SCORTA

      U     "CLOCK 0,1 s";
      UN    "CLOCK 0,1 s";
      =     "A      51.5";
NETWORK
TITLE =SCORTA

      U     "CLOCK 0,1 s";
      UN    "CLOCK 0,1 s";
      =     "A      51.6";
NETWORK
TITLE =SCORTA

      U     "CLOCK 0,1 s";
      UN    "CLOCK 0,1 s";
      =     "A      51.7";
NETWORK
TITLE =VELOCITA' INVERTER CATENE - USCITA ANALOGICA

      L     "DB DATI".VCI;
      T     "C.VC";

END_FUNCTION

